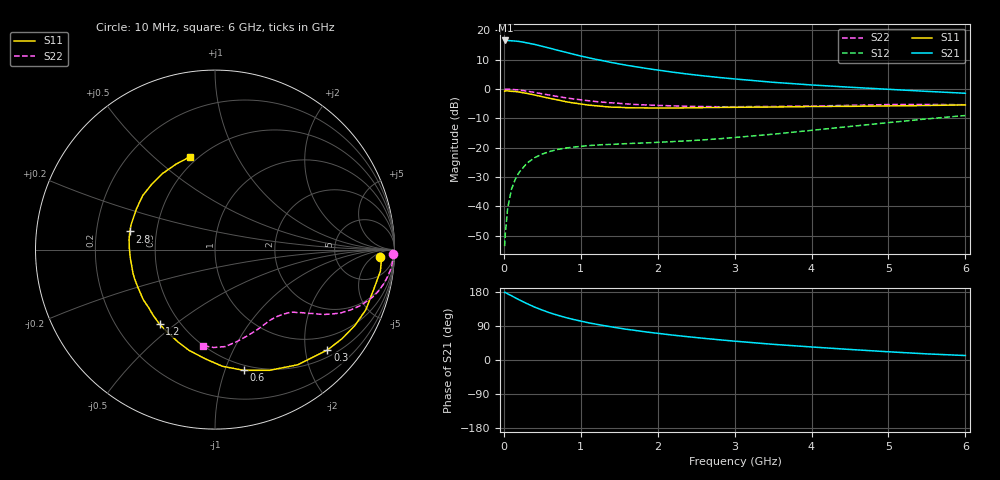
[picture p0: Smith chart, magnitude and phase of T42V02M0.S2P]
! Infineon Technologies  Discrete & RF Semiconductors
! BFR182T
! Si NPN RF Bipolar Junction Transistor in SC75
! VCE = 2 V  IC = 2 mA
! Common Emitter S-Parameters:  October  1999
# GHz  S  MA  R  50
!  f  S11  S21  S12  S22
! GHz  MAG  ANG  MAG  ANG  MAG  ANG  MAG  ANG
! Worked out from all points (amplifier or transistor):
!   36 points, 10 MHz to 6 GHz, reference 50 ohm
!   highest |S21| = 16.5 dB at 20 MHz (marker M1)
!   |S21| within 3 dB of that: start of sweep to 650 MHz
!   unconditionally stable (mu >= 1): 1.96 GHz to 4.362 GHz
!   at 250 MHz: K = 0.14, MSG = 21.4 dB, |S12| = -26.8 dB
!   at 1.4 GHz: K = 0.79, MSG = 14.0 dB, |S12| = -18.9 dB
!   at 6 GHz: K = 0.84, MSG = 3.8 dB, |S12| = -9.0 dB
!   lowest NFmin = 1.10 dB at 450 MHz
!   S11 on the Smith chart (normalised r, x): 10 MHz: 19, -9; 300 MHz: 0.65, -2.47; 600 MHz: 0.45, -1.16; 1.2 GHz: 0.39, -0.44; 2.8 GHz: 0.35, +0.09; 6 GHz: 0.46, +0.66
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0.01  0.9178 -2.5  6.667 178.4  0.0021 80.5  0.9903 -1.3
0.02  0.9305 -1.6  6.713 178.2  0.0035 94.9  0.9892 -1.2
0.05  0.9293 -7.4  6.701 174.6  0.0094 87.9  0.9932 -3.0
0.1  0.9117 -14.0  6.622 169.6  0.0197 82.8  0.9871 -6.0
0.2  0.8864 -28.6  6.452 158.7  0.0382 74.9  0.9589 -11.5
0.3  0.8398 -41.8  6.111 148.9  0.0545 68.0  0.9201 -16.5
0.4  0.7901 -54.3  5.744 139.6  0.0675 60.9  0.8734 -20.7
0.5  0.7384 -65.6  5.333 131.7  0.078 56.2  0.8282 -23.9
0.6  0.6913 -76.7  4.941 124.3  0.0865 52.2  0.7849 -26.7
0.8  0.6099 -95.4  4.241 112.3  0.0985 46.4  0.7097 -30.6
0.9  0.5794 -104.5  3.924 107.2  0.102 44.1  0.6783 -32.0
1.1  0.5314 -119.8  3.414 98.2  0.1086 41.4  0.631 -34.3
1.2  0.5177 -126.6  3.192 94.5  0.1106 40.6  0.6107 -35.3
1.4  0.4908 -139.1  2.825 87.4  0.1136 39.7  0.5814 -37.2
1.6  0.4803 -150.7  2.531 81.0  0.1174 39.7  0.5564 -38.8
1.9  0.4754 -164.0  2.192 72.8  0.1217 41.2  0.5316 -42.1
2.2  0.4744 -174.9  1.933 65.6  0.1272 43.5  0.5163 -45.0
2.8  0.4852 168.0  1.57 53.4  0.1419 49.0  0.4983 -52.6
3.5  0.4932 152.5  1.301 41.4  0.1698 54.8  0.5042 -61.9
4.5  0.5064 134.3  1.072 27.8  0.23 58.1  0.5266 -76.5
5.5  0.5234 114.5  0.911 16.1  0.3096 56.0  0.5454 -90.7
6  0.536 104.8  0.846 11.8  0.3536 53.0  0.5395 -97.2
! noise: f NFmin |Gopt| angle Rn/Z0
0.45  1.1  0.42  29  0.36
0.9  1.2  0.4  58  0.3
1.8  1.85  0.32  126  0.22
